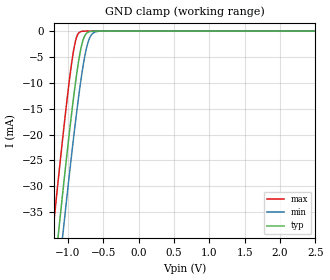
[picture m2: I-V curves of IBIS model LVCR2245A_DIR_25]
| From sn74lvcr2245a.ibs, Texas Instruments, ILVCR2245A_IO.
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[Model]   LVCR2245A_DIR_25
Model_type  Input
Vinl=0.7
Vinh=1.7
| variable   typ   min   max
C_comp   3.49pF   3.15pF   4.12pF
[Temperature Range]   40   100   -40
| Ambient temperature   25   85   -40
[Voltage range]   2.5   2.3   2.7
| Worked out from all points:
|   GND clamp passes 1 mA (typ) near -0.77 V on its own axis
[GND Clamp]
| LVCR2245A_DIR_25
|   Voltage   I(typ)   I(min)   I(max)
-5.5V     -655.9mA   -662.8mA   -647.2mA
-1.215V   -49.64mA   -57.94mA   -39mA
-1.14V    -39.76mA   -48.06mA   -29.1mA
-1.12V    -37.16mA   -45.45mA   -26.51mA
-1.08V    -32.01mA   -40.28mA   -21.4mA
-1.06V    -29.47mA   -37.73mA   -18.9mA
-960mV    -17.27mA   -25.29mA   -7.384mA
-890mV    -9.607mA   -17.12mA   -1.735mA
-785mV    -1.672mA   -6.641mA   -21.69uA
-720mV    -242.7uA   -2.356mA   -1.024uA
-650mV    -22.03uA   -444.3uA   -37.97nA
2.5V      4.713pA    7.579pA    4.389pA
